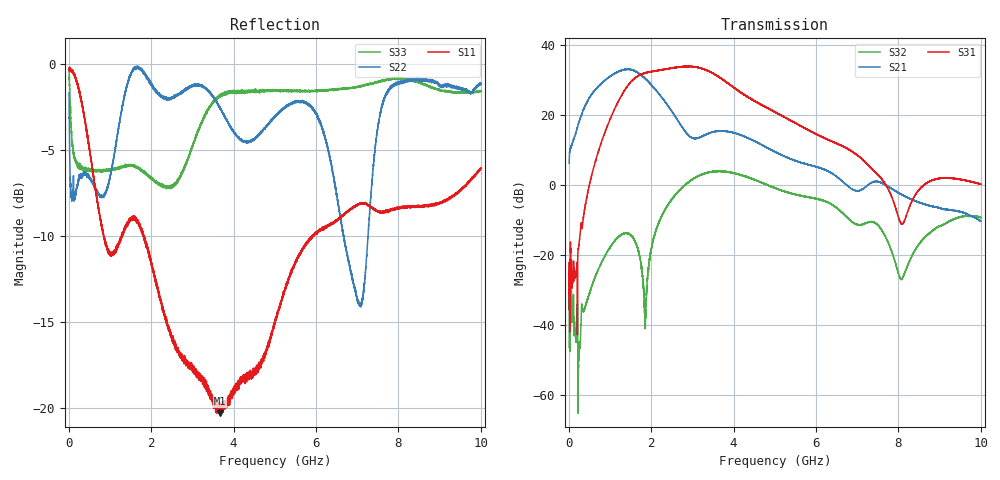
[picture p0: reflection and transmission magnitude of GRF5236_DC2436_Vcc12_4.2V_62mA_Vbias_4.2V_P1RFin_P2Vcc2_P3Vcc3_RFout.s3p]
!Keysight Technologies,N5245B,MY56052315,A.20.20.05
!Date: Friday, August 21, 2026 13:51:08
!Correction: S11(C  3-Port  )
!S12(C  3-Port  )
!S13(C  3-Port  )
!S21(C  3-Port  )
!S22(C  3-Port  )
!S23(C  3-Port  )
!S31(C  3-Port  )
!S32(C  3-Port  )
!S33(C  3-Port  )
!S3P File: Measurements: <S11,S12,S13>,
!<S21,S22,S23>,
!<S31,S32,S33>:
# Hz S  RI  R 50
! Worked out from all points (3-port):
!   9991 points, 10 MHz to 10 GHz, reference 50 ohm
!   strongest paths, dB at 10 MHz, 2.507 GHz, 5.005 GHz, 7.503 GHz, 10 GHz:
!     S31: -29.0, 33.4, 20.8, 2.8, 0.2
!     S21: 6.1, 20.9, 9.4, 0.9, -10.4
!     S32: -35.7, -4.1, -0.9, -11.5, -9.4
!   lowest |S11| = -20.3 dB at 3.659 GHz (marker M1), VSWR 1.21, Z = 52.3 + j9.63 ohm
!   |S11| at or under -10 dB: 847.2 MHz to 1.283 GHz (436.1 MHz wide, 40.9 % of centre); 1.823 GHz to 5.911 GHz (4.088 GHz wide, 106 % of centre); 5.924176 GHz to 5.92962 GHz (5.444 MHz wide, 0.0919 % of centre)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
1e7  0.9579 -0.0286  -1.47e-05 -0.00133  -0.00165 0.000113
     0.6677 1.91  0.5064 -0.6506  -0.000783 -0.000545
     -0.0084 -0.0346  0.0148 0.00705  0.8968 -0.3591
6.13e8  0.0323 -0.4632  -0.0019 0.00788  -0.000246 0.000383
        19.35 9.793  -0.4296 0.0934  0.00378 -0.00625
        1.794 0.2358  0.0436 0.00598  -0.4853 -0.0698
1.105e9  -0.0529 -0.2771  0.000921 0.0116  -2e-05 0.000857
         34.13 -18.19  -0.5231 -0.1563  -0.0147 -0.0191
         7.882 -8.845  0.0926 -0.1247  -0.4918 -0.0348
1.516e9  -0.2581 -0.2366  0.000711 0.0157  -1.94e-05 0.00141
         1.882 -43.72  -0.9296 -0.0751  -0.0395 0.00791
         -11.77 -27.44  -0.087 -0.1664  -0.5076 -0.00956
2.041e9  -0.2186 0.1315  0.00403 0.0202  0.000574 0.00132
         -23.3 -10.11  -0.7506 0.4183  -0.00652 0.0307
         -40.97 8.922  0.1379 -0.0652  -0.4611 0.00499
2.811e9  0.0288 0.1332  0.0032 0.0224  0.000835 0.00117
         -5.795 1.303  -0.6334 0.55  -0.00496 0.0175
         6.483 48.43  -0.2694 -0.9461  -0.4843 -0.1301
3.249e9  0.0612 0.1027  0.00107 0.0264  0.000604 0.00189
         -4.829 -1.02  -0.627 0.5848  -0.0049 0.03
         38.94 23.69  -1.265 -0.6297  -0.6719 -0.1325
3.659e9  0.0309 0.0912  0.000181 0.0322  0.000749 0.00167
         -5.852 0.0326  -0.51 0.5452  0.011 0.0368
         33.3 -7.675  -1.494 0.4305  -0.8023 0.0294
5.005e9  -0.1437 0.1016  0.0102 0.0418  0.000783 0.00245
         -1.553 2.523  -0.2718 0.6474  0.0269 0.00693
         -1.573 -10.85  0.3057 0.851  -0.7857 0.2798
1e10  -0.0969 0.4878  0.0345 0.0333  0.000484 0.000679
      0.1989 0.228  -0.1021 0.8705  0.0239 0.00221
      -0.8772 0.5168  0.3333 -0.0625  0.2923 0.7826
